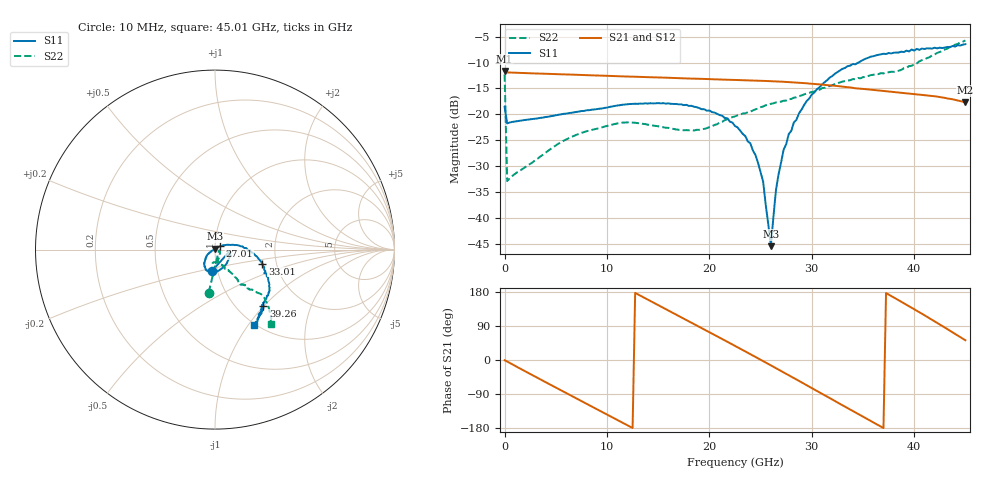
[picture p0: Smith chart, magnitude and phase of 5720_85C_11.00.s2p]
! Device:  ADRF5720
! Description: 0.5dB LSB GaAs MMIC 6-bit Digital Attenuator
! Frequency:  0.000009 -  40 GHz
! Ports:
!	RF1	= Port 1
!	RF2	= Port 2
! Vdd:  3.3 Volt
! Vss:  -3.3 Volt
! Control:  0/3.3 Volt
! State:  11.00 dB attenuation
! Data:  The device was measured using G-S-G Probes on a matrix board.
!  Data was collected using an calibrated 4 port network analyzer.
!  The reference plane for this measurement is at the launchers.
! Note:  Analog Devices supplies this data as a sample of measured data
!  for this product.  Your particular data for this product may vary.
!  Data was taken at 85 degrees C.
!  Analog Devices reserves the right to change this data at anytime.
# GHZ S DB R 45.0
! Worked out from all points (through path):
!   181 points, 10 MHz to 45.01 GHz, reference 45 ohm
!   highest |S21| = -11.62 dB at 10 MHz (marker M1); lowest = -17.7 dB at 45.01 GHz (marker M2)
!   group delay of S21, straight-line fit = 40.8 ps
!   lowest |S11| = -45.5 dB at 26.01 GHz (marker M3), VSWR 1.01, Z = 45.1 + j0.473 ohm
!   |S11| at or under -10 dB: start of sweep to 34.56 GHz
!   |S22| runs from -32.9 to -5.7 dB; largest |S21 - S12| = 0.0014
!   S11 on the Smith chart (normalised r, x): 10 MHz: 0.94, -0.22; 27.01 GHz: 1.06, +0.04; 33.01 GHz: 1.69, -0.28; 39.26 GHz: 1.31, -0.99; 45.01 GHz: 0.98, -1.07
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0.01  -18.55 -97.5  -11.62 -0.8  -11.61 -0.8  -12.30 -98.5
0.26  -21.76 -7.4  -11.91 -4.0  -11.91 -4.0  -32.91 -20.6
4.26  -20.48 -38.4  -12.19 -62.0  -12.18 -62.0  -27.06 -57.4
7.76  -19.35 -63.2  -12.42 -112.0  -12.41 -111.9  -23.45 -79.0
11.51  -18.16 -85.1  -12.67 -165.2  -12.67 -165.1  -21.62 -94.6
15.26  -17.89 -103.4  -12.90 141.4  -12.89 141.5  -22.43 -99.6
19.01  -18.79 -118.9  -13.14 87.8  -13.13 88.0  -23.02 -81.3
22.76  -22.55 -134.5  -13.38 33.6  -13.38 33.9  -20.22 -64.9
24.01  -25.63 -145.2  -13.46 15.4  -13.46 15.6  -19.48 -63.2
24.76  -29.40 -153.2  -13.51 4.5  -13.51 4.7  -18.89 -62.4
25.26  -33.03 -161.0  -13.55 -2.9  -13.54 -2.7  -18.49 -61.7
26.01  -45.50 81.3  -13.60 -14.1  -13.59 -13.8  -17.98 -60.4
26.51  -34.67 43.2  -13.64 -21.6  -13.64 -21.2  -17.71 -59.1
27.01  -29.35 36.1  -13.69 -29.0  -13.68 -28.7  -17.56 -58.0
27.26  -26.83 26.7  -13.72 -32.8  -13.72 -32.5  -17.39 -58.2
28.26  -21.56 18.9  -13.85 -47.8  -13.84 -47.5  -16.79 -56.8
30.26  -15.80 3.2  -14.14 -77.9  -14.13 -77.6  -15.62 -54.5
33.01  -11.21 -16.4  -14.66 -119.6  -14.65 -119.2  -13.68 -53.3
37.76  -8.24 -41.7  -15.64 168.9  -15.63 169.3  -11.77 -50.3
39.26  -7.69 -49.3  -15.96 145.8  -15.94 146.2  -11.01 -50.0
42.26  -7.26 -55.2  -16.59 97.9  -16.57 98.3  -8.13 -44.5
45.01  -6.44 -62.5  -17.69 52.0  -17.67 52.4  -5.73 -52.9
